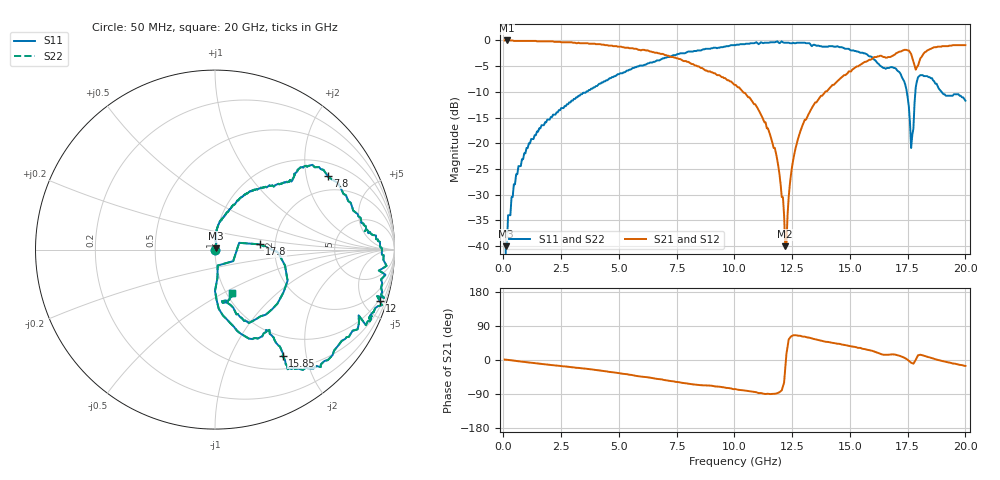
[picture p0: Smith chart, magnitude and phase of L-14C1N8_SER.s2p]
# MHZ S MA R 50
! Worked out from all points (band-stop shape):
!   400 points, 50 MHz to 20 GHz, reference 50 ohm
!   highest |S21| = 0.00 dB at 150 MHz (marker M1); lowest = -40.0 dB at 12.2 GHz (marker M2)
!   |S21| within 3 dB of the highest: start of sweep to 7.16 GHz; 18.13 GHz to end of sweep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
!   lowest |S11| = -40.0 dB at 100 MHz (marker M3), VSWR 1.02, Z = 50.7 + j0.729 ohm
!   |S11| at or under -10 dB: start of sweep to 3.581 GHz; 17.46 GHz to 17.83 GHz (371.9 MHz wide, 2.11 % of centre); 18.97 GHz to end of sweep
!   |S22| runs from - to -0.2 dB; largest |S21 - S12| = 0
!   S11 on the Smith chart (normalised r, x): 50 MHz: 1.00, +0.00; 7.8 GHz: 1.42, +2.67; 12 GHz: 0.90, -6.49; 15.85 GHz: 0.69, -1.60; 17.8 GHz: 1.66, +0.10; 20 GHz: 1.07, -0.55
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50  0 19.6  1 1.1  1 1.1  0 19.6
100  0.01 46.0  1 0.9  1 0.9  0.01 46.0
150  0.01 72.4  1 0.6  1 0.6  0.01 72.4
200  0.02 75.0  1 0.2  1 0.2  0.02 75.0
450  0.04 77.7  0.99 -1.5  0.99 -1.5  0.04 77.7
1100  0.1 85.7  0.99 -6.5  0.99 -6.5  0.1 85.7
3400  0.3 65.1  0.94 -22.1  0.94 -22.1  0.3 65.1
6700  0.64 43.9  0.75 -50.2  0.75 -50.2  0.64 43.9
7800  0.75 33.3  0.63 -60.7  0.63 -60.7  0.75 33.3
10050  0.9 3.7  0.37 -76.8  0.37 -76.8  0.9 3.7
11350  0.95 -12.4  0.16 -89.7  0.16 -89.7  0.95 -12.4
12000  0.96 -17.2  0.04 -82.5  0.04 -82.5  0.96 -17.2
12200  0.95 -20.8  0.01 -22.4  0.01 -22.4  0.95 -20.8
12550  0.95 -23.0  0.07 65.3  0.07 65.3  0.95 -23.0
13350  0.88 -24.6  0.22 57.0  0.22 57.0  0.88 -24.6
15850  0.7 -57.5  0.65 25.9  0.65 25.9  0.7 -57.5
16700  0.54 -59.9  0.69 14.1  0.69 14.1  0.54 -59.9
17400  0.37 -83.1  0.81 4.4  0.81 4.4  0.37 -83.1
17650  0.09 -80.4  0.74 -7.3  0.74 -7.3  0.09 -80.4
17800  0.25 6.7  0.57 -4.8  0.57 -4.8  0.25 6.7
18350  0.45 -65.3  0.8 8.2  0.8 8.2  0.45 -65.3
20000  0.26 -68.0  0.9 -15.6  0.9 -15.6  0.26 -68.0
